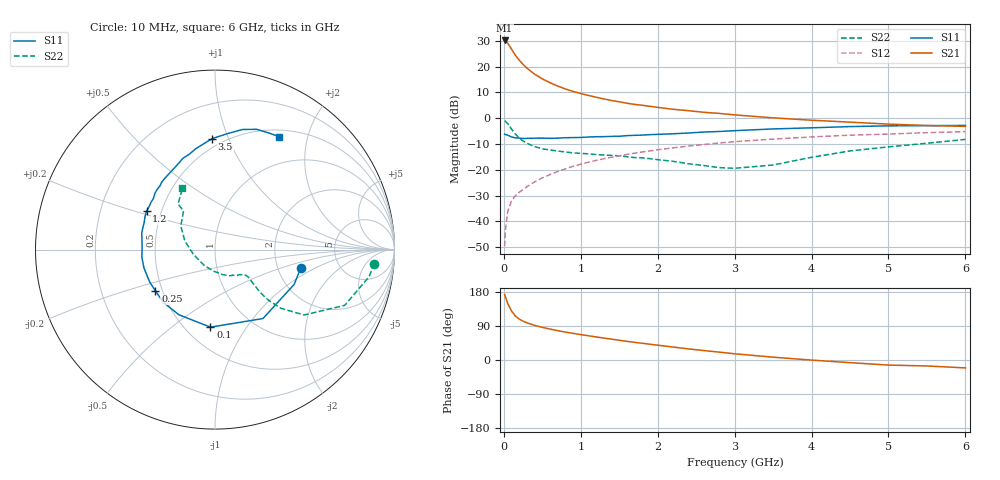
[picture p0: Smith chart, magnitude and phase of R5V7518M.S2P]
! SIEMENS Small Signal Semiconductors
! BFR183
! Si NPN RF Bipolar Junction Transistor in SOT23
! VCE = 0.75 V  IC = 18 mA
! Common Emitter S-Parameters:  May  1996
# GHz  S  MA  R  50
!  f  S11  S21  S12  S22
! GHz  MAG  ANG  MAG  ANG  MAG  ANG  MAG  ANG
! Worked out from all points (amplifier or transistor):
!   36 points, 10 MHz to 6 GHz, reference 50 ohm
!   highest |S21| = 30.1 dB at 10 MHz (marker M1)
!   |S21| within 3 dB of that: start of sweep to 92.11 MHz
!   unconditionally stable (mu >= 1): 377.3 MHz to 3.336 GHz
!   at 250 MHz: K = 0.88, MSG = 24.2 dB, |S12| = -27.6 dB
!   at 1.4 GHz: K = 1.12, MAG = 8.9 dB, |S12| = -15.1 dB
!   at 6 GHz: K = 0.99, MSG = 1.0 dB, |S12| = -5.2 dB
!   S11 on the Smith chart (normalised r, x): 10 MHz: 2.69, -0.73; 100 MHz: 0.66, -0.70; 250 MHz: 0.46, -0.25; 1.2 GHz: 0.41, +0.22; 3.5 GHz: 0.44, +0.87; 6 GHz: 0.59, +1.55
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0.01  0.4888 -12.2  32.1 173.3  0.0033 82.9  0.8914 -5.0
0.02  0.4816 -23.8  31.72 166.5  0.0066 79.3  0.8714 -10.0
0.05  0.4679 -55.2  28.49 149.3  0.0155 71.5  0.7863 -23.3
0.1  0.4328 -93.4  21.79 129.2  0.0249 62.4  0.6154 -36.3
0.15  0.415 -118.9  16.64 116.1  0.0315 60.0  0.4914 -41.7
0.2  0.4112 -134.1  13.35 108.1  0.0365 60.4  0.4113 -43.4
0.25  0.404 -145.2  10.99 102.4  0.0415 61.0  0.3605 -43.5
0.3  0.4063 -153.9  9.313 98.0  0.0471 62.6  0.3265 -43.0
0.4  0.4089 -165.7  7.141 91.5  0.0581 64.9  0.2807 -41.5
0.5  0.4098 -174.2  5.783 86.2  0.0694 66.1  0.2545 -40.2
0.6  0.4062 179.0  4.867 81.6  0.081 66.3  0.2416 -39.5
0.8  0.418 167.6  3.685 73.7  0.1044 66.1  0.2209 -40.0
0.9  0.4202 163.3  3.296 70.3  0.1169 65.7  0.2122 -40.5
1.1  0.431 154.9  2.755 64.0  0.1401 64.4  0.2033 -43.6
1.2  0.4369 150.7  2.547 60.8  0.1519 63.5  0.1971 -45.0
1.6  0.4588 136.9  1.948 49.2  0.1981 59.1  0.1786 -53.5
2.2  0.4984 119.6  1.486 34.2  0.2663 51.4  0.1456 -73.3
3  0.5724 100.8  1.159 16.4  0.35 39.9  0.1067 -124.2
3.5  0.6184 91.5  1.014 7.4  0.3936 32.5  0.1236 -167.8
4.5  0.6866 77.1  0.837 -7.0  0.4689 18.7  0.2317 145.4
5.5  0.716 65.1  0.721 -15.7  0.5241 7.0  0.3264 129.1
6  0.7229 60.5  0.693 -20.9  0.5478 -0.4  0.3875 117.9
